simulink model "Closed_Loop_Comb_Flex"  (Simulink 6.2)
settings: Solver=ode45  StartTime=0.0  StopTime=40  RelTol=1e-3
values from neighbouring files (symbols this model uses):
  d2r = pi/180    (= 0.0174532925199)    [run.m]    (also in init.m)
undefined symbols (not defined in the file or in its folder): Ac, Bc, Cc, Dc

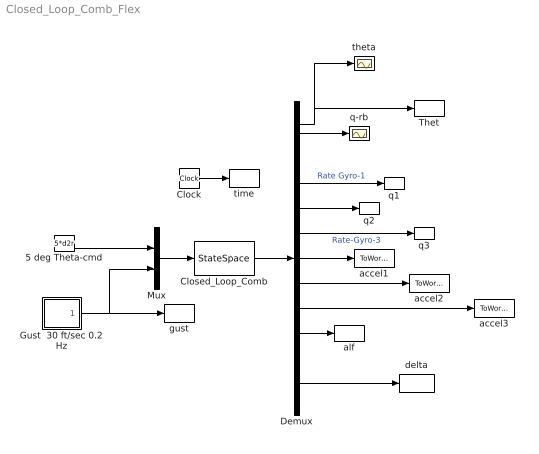
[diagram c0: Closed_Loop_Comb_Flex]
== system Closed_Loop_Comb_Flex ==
  5 deg Theta-cmd : Constant  Value=5*d2r
  Clock : Clock
  Closed_Loop_Comb : StateSpace  A=Ac  B=Bc  C=Cc  D=Dc
  Demux : Demux  Outputs=13
  Gust  30 ft/sec 0.2 Hz : Subsystem
  Mux : Mux  Inputs=2
  Thet : ToWorkspace  VariableName=theta  SampleTime=-1  SaveFormat=Array
  accel1 : ToWorkspace  VariableName=accel1  SampleTime=-1  SaveFormat=Array
  accel2 : ToWorkspace  VariableName=accel2  SampleTime=-1  SaveFormat=Array
  accel3 : ToWorkspace  VariableName=accel3  SampleTime=-1  SaveFormat=Array
  alf : ToWorkspace  VariableName=alpha  SampleTime=-1  SaveFormat=Array
  delta : ToWorkspace  VariableName=delta  SampleTime=-1  SaveFormat=Array
  gust : ToWorkspace  VariableName=Gust  SampleTime=-1  SaveFormat=Array
  q-rb : Scope
  q1 : ToWorkspace  VariableName=q1  SampleTime=-1  SaveFormat=Array
  q2 : ToWorkspace  VariableName=q2  SampleTime=-1  SaveFormat=Array
  q3 : ToWorkspace  VariableName=q3  SampleTime=-1  SaveFormat=Array
  theta : Scope
  time : ToWorkspace  VariableName=time  SampleTime=-1  SaveFormat=Array
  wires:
  Mux/1 -> Closed_Loop_Comb/1
  Closed_Loop_Comb/1 -> Demux/1
  5 deg Theta-cmd/1 -> Mux/1
  Demux/2 -> q-rb/1
  Demux/1 -> theta/1, Thet/1
  Gust  30 ft/sec 0.2 Hz/1(Vgust) -> Mux/2, gust/1
  Clock/1 -> time/1
  Demux/12 -> delta/1
  Demux/4 -> q1/1  "Rate Gyro-1"
  Demux/5 -> q2/1
  Demux/6 -> q3/1  "Rate-Gyro-3"
  Demux/10 -> alf/1
  Demux/7 -> accel1/1
  Demux/8 -> accel2/1
  Demux/9 -> accel3/1

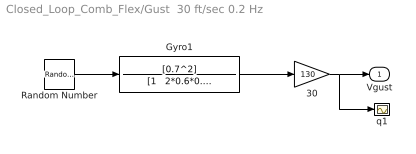
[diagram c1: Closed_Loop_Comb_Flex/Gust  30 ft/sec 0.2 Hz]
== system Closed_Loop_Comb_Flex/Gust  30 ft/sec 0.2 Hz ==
  30 : Gain  Gain=130
  Gyro1 : TransferFcn  Numerator=[0.7^2]  Denominator="[1   2*0.6*0.7   0.7^2]"
  Random Number : RandomNumber  Seed=-2  SampleTime=0
  q1 : Scope
  Vgust : Outport
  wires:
  30/1 -> q1/1, Vgust/1
  Gyro1/1 -> 30/1
  Random Number/1 -> Gyro1/1
